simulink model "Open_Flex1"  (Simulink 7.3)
settings: Solver=ode4  StartTime=0.0  StopTime=20  RelTol=1e-3
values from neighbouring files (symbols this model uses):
  Ts = 0.04    [run.m]    (also in z2s_transf.m)
undefined symbols (not defined in the file or in its folder): Acts, Afls, Alfc, Apfc, Asz, Bcts, Bfls, Blfc, Bpfc, Bsz, Ccts, Cfls, Clfc, Cpfc, Csz, Dcts, Dfls, Dlfc, Dpfc, Dsz, TVC

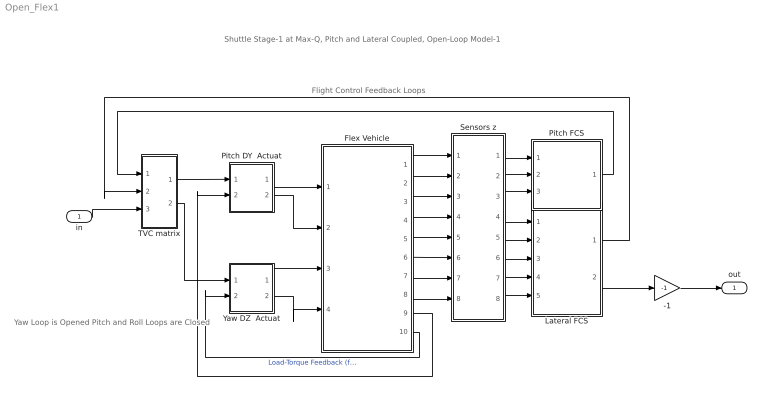
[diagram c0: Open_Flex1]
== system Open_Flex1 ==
  note: Shuttle Stage-1 at Max-Q, Pitch and Lateral Coupled, Open-Loop Model-1
  note: Yaw Loop is Opened Pitch and Roll Loops are Closed
  note: Flight Control Feedback Loops
  in : Inport  OutDataType=sfix(16)  OutScaling=2^0
  -1 : Gain  Gain=-1  ParameterDataType=sfix(16)  ParameterScaling=2^0  OutDataType=sfix(16)  OutScaling=2^0
  Flex Vehicle : Subsystem
  Lateral FCS : Subsystem
  Pitch DY  Actuat : Subsystem
  Pitch FCS : Subsystem
  Sensors z : Subsystem
  TVC matrix : Subsystem
  Yaw DZ  Actuat : Subsystem
  out : Outport  OutDataType=sfix(16)  OutScaling=2^0
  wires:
  TVC matrix/1(dy) -> Pitch DY  Actuat/1(dyc)
  TVC matrix/2(dz) -> Yaw DZ  Actuat/1(dzc)
  Pitch DY  Actuat/1(dy) -> Flex Vehicle/1(dy)
  Yaw DZ  Actuat/1(dz) -> Flex Vehicle/3(dz)
  Pitch DY  Actuat/2(dydd) -> Flex Vehicle/2(dydd)
  Yaw DZ  Actuat/2(dzdd) -> Flex Vehicle/4(dzdd)
  -1/1 -> out/1
  Flex Vehicle/10(TLz) -> Yaw DZ  Actuat/2(TLz)  "Load-Torque Feedback (ft-lb)"
  Flex Vehicle/9(TLy) -> Pitch DY  Actuat/2(TLy)
  Flex Vehicle/1(theta) -> Sensors z/1(thei)
  Sensors z/1(theo) -> Pitch FCS/1(theta)
  Flex Vehicle/2(q-flx) -> Sensors z/2(qi)
  Sensors z/2(qo) -> Pitch FCS/2(q)
  Flex Vehicle/3(Nz) -> Sensors z/3(Nzi)
  Sensors z/3(Nzo) -> Pitch FCS/3(Nz)
  Flex Vehicle/4(phi) -> Sensors z/4(phi)
  Sensors z/4(pho) -> Lateral FCS/1(phi-er)
  Flex Vehicle/5(psi) -> Sensors z/5("psi ")
  Sensors z/5(pso) -> Lateral FCS/2(psi-er)
  Flex Vehicle/6(p-flx) -> Sensors z/6(pi)
  Sensors z/6(po) -> Lateral FCS/3(p)
  Flex Vehicle/7(r-flx) -> Sensors z/7(ri)
  Sensors z/7(ro) -> Lateral FCS/4(r)
  Flex Vehicle/8(Ny) -> Sensors z/8(Nyi)
  Sensors z/8(Nyo) -> Lateral FCS/5(Ny)
  Lateral FCS/1(DP_TVC) -> TVC matrix/2(roll)
  in/1 -> TVC matrix/3(yaw)
  Lateral FCS/2(DR_TVC) -> -1/1
  Pitch FCS/1(DQ_TVC) -> TVC matrix/1(ptch)

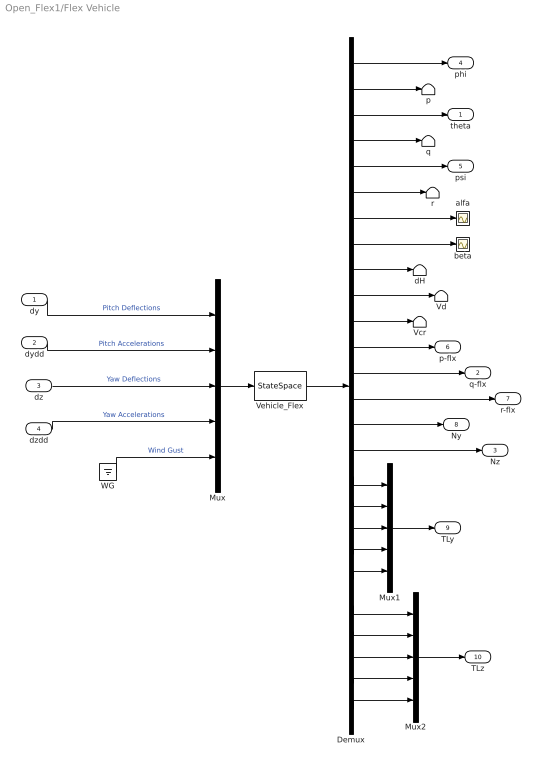
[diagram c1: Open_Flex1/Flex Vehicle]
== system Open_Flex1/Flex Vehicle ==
  dy : Inport  PortDimensions=5  OutDataType=sfix(16)  OutScaling=2^0
  dydd : Inport  Port=2  PortDimensions=5  OutDataType=sfix(16)  OutScaling=2^0
  dz : Inport  Port=3  PortDimensions=5  OutDataType=sfix(16)  OutScaling=2^0
  dzdd : Inport  Port=4  PortDimensions=5  OutDataType=sfix(16)  OutScaling=2^0
  Demux : Demux  Outputs=26
  Mux : Mux  Inputs="[5  5  5  5  1]"
  Mux1 : Mux  Inputs=5
  Mux2 : Mux  Inputs=5
  Vcr : Terminator
  Vd : Terminator
  Vehicle_Flex : StateSpace  A=Afls  B=Bfls  C=Cfls  D=Dfls
  WG : Ground
  alfa : Scope
  beta : Scope
  dH : Terminator
  p : Terminator
  q : Terminator
  r : Terminator
  theta : Outport  OutDataType=sfix(16)  OutScaling=2^0
  q-flx : Outport  Port=2  OutDataType=sfix(16)  OutScaling=2^0
  Nz : Outport  Port=3  OutDataType=sfix(16)  OutScaling=2^0
  phi : Outport  Port=4  OutDataType=sfix(16)  OutScaling=2^0
  psi : Outport  Port=5  OutDataType=sfix(16)  OutScaling=2^0
  p-flx : Outport  Port=6  OutDataType=sfix(16)  OutScaling=2^0
  r-flx : Outport  Port=7  OutDataType=sfix(16)  OutScaling=2^0
  Ny : Outport  Port=8  OutDataType=sfix(16)  OutScaling=2^0
  TLy : Outport  Port=9  OutDataType=sfix(16)  OutScaling=2^0
  TLz : Outport  Port=10  OutDataType=sfix(16)  OutScaling=2^0
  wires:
  Mux/1 -> Vehicle_Flex/1
  WG/1 -> Mux/5  "Wind Gust"
  dz/1 -> Mux/3  "Yaw Deflections"
  dydd/1 -> Mux/2  "Pitch Accelerations"
  dy/1 -> Mux/1  "Pitch Deflections"
  Demux/1 -> phi/1
  Demux/5 -> psi/1
  Demux/2 -> p/1
  Demux/6 -> r/1
  Demux/8 -> beta/1
  Demux/12 -> p-flx/1
  Demux/13 -> q-flx/1
  Demux/15 -> Ny/1
  Demux/3 -> theta/1
  Demux/4 -> q/1
  Demux/7 -> alfa/1
  Demux/11 -> Vcr/1
  Demux/10 -> Vd/1
  Demux/9 -> dH/1
  Demux/14 -> r-flx/1
  Demux/16 -> Nz/1
  dzdd/1 -> Mux/4  "Yaw Accelerations"
  Vehicle_Flex/1 -> Demux/1
  Demux/21 -> Mux1/5
  Demux/20 -> Mux1/4
  Demux/19 -> Mux1/3
  Demux/18 -> Mux1/2
  Demux/17 -> Mux1/1
  Demux/22 -> Mux2/1
  Demux/23 -> Mux2/2
  Demux/24 -> Mux2/3
  Demux/25 -> Mux2/4
  Demux/26 -> Mux2/5
  Mux1/1 -> TLy/1
  Mux2/1 -> TLz/1

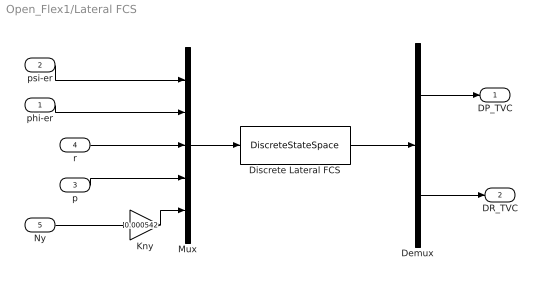
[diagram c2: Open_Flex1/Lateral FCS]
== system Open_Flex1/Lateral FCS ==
  phi-er : Inport  OutDataType=sfix(16)  OutScaling=2^0
  psi-er : Inport  Port=2  OutDataType=sfix(16)  OutScaling=2^0
  p : Inport  Port=3  OutDataType=sfix(16)  OutScaling=2^0
  r : Inport  Port=4  OutDataType=sfix(16)  OutScaling=2^0
  Ny : Inport  Port=5  OutDataType=sfix(16)  OutScaling=2^0
  Demux : Demux  Outputs=2
  Discrete Lateral FCS : DiscreteStateSpace  A=Alfc  B=Blfc  C=Clfc  D=Dlfc  SampleTime=Ts
  Kny : Gain  Gain=0.000542  ParameterDataType=sfix(16)  ParameterScaling=2^0  OutDataType=sfix(16)  OutScaling=2^0
  Mux : Mux  Inputs=5
  DP_TVC : Outport  OutDataType=sfix(16)  OutScaling=2^0
  DR_TVC : Outport  Port=2  OutDataType=sfix(16)  OutScaling=2^0
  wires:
  psi-er/1 -> Mux/1
  phi-er/1 -> Mux/2
  r/1 -> Mux/3
  Mux/1 -> Discrete Lateral FCS/1
  Discrete Lateral FCS/1 -> Demux/1
  Demux/1 -> DP_TVC/1
  Demux/2 -> DR_TVC/1
  p/1 -> Mux/4
  Ny/1 -> Kny/1
  Kny/1 -> Mux/5

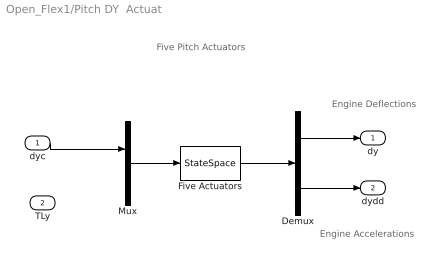
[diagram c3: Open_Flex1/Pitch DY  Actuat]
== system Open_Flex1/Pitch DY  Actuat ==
  note: Engine Accelerations
  note: Engine Deflections
  note: Five Pitch Actuators
  dyc : Inport  OutDataType=sfix(16)  OutScaling=2^0
  TLy : Inport  Port=2  OutDataType=sfix(16)  OutScaling=2^0
  Demux : Demux  Outputs=[5, 5]
  Five Actuators : StateSpace  A=Acts  B=Bcts  C=Ccts  D=Dcts
  Mux : Mux  Inputs="[5  5]"
  dy : Outport  OutDataType=sfix(16)  OutScaling=2^0
  dydd : Outport  Port=2  OutDataType=sfix(16)  OutScaling=2^0
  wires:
  Mux/1 -> Five Actuators/1
  dyc/1 -> Mux/1
  Five Actuators/1 -> Demux/1
  Demux/1 -> dy/1
  Demux/2 -> dydd/1

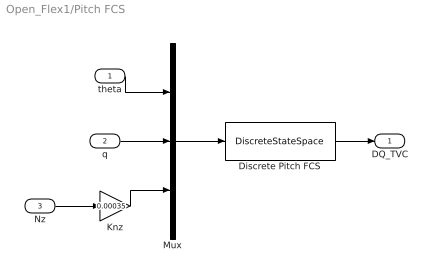
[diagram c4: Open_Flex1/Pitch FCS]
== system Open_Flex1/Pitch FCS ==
  theta : Inport  OutDataType=sfix(16)  OutScaling=2^0
  q : Inport  Port=2  OutDataType=sfix(16)  OutScaling=2^0
  Nz : Inport  Port=3  OutDataType=sfix(16)  OutScaling=2^0
  Discrete Pitch FCS : DiscreteStateSpace  A=Apfc  B=Bpfc  C=Cpfc  D=Dpfc  SampleTime=Ts
  Knz : Gain  Gain=0.00035  ParameterDataType=sfix(16)  ParameterScaling=2^0  OutDataType=sfix(16)  OutScaling=2^0
  Mux : Mux  Inputs=3
  DQ_TVC : Outport  OutDataType=sfix(16)  OutScaling=2^0
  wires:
  Mux/1 -> Discrete Pitch FCS/1
  Nz/1 -> Knz/1
  q/1 -> Mux/2
  theta/1 -> Mux/1
  Discrete Pitch FCS/1 -> DQ_TVC/1
  Knz/1 -> Mux/3

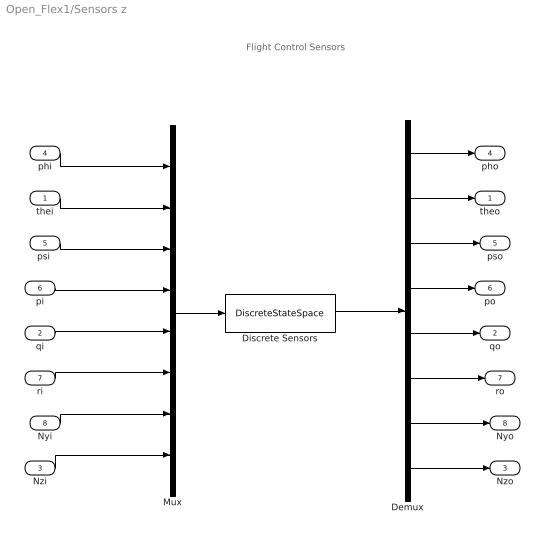
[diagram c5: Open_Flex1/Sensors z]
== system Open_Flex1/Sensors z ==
  note: Flight Control Sensors
  thei : Inport  PortDimensions=1  OutDataType=sfix(16)  OutScaling=2^0
  qi : Inport  Port=2  PortDimensions=1  OutDataType=sfix(16)  OutScaling=2^0
  Nzi : Inport  Port=3  PortDimensions=1  OutDataType=sfix(16)  OutScaling=2^0
  phi : Inport  Port=4  PortDimensions=1  OutDataType=sfix(16)  OutScaling=2^0
  "psi " : Inport  Port=5  PortDimensions=1  OutDataType=sfix(16)  OutScaling=2^0
  pi : Inport  Port=6  PortDimensions=1  OutDataType=sfix(16)  OutScaling=2^0
  ri : Inport  Port=7  PortDimensions=1  OutDataType=sfix(16)  OutScaling=2^0
  Nyi : Inport  Port=8  PortDimensions=1  OutDataType=sfix(16)  OutScaling=2^0
  Demux : Demux  Outputs=8
  Discrete Sensors : DiscreteStateSpace  A=Asz  B=Bsz  C=Csz  D=Dsz  SampleTime=Ts
  Mux : Mux  Inputs=8
  theo : Outport  OutDataType=sfix(16)  OutScaling=2^0
  qo : Outport  Port=2  OutDataType=sfix(16)  OutScaling=2^0
  Nzo : Outport  Port=3  OutDataType=sfix(16)  OutScaling=2^0
  pho : Outport  Port=4  OutDataType=sfix(16)  OutScaling=2^0
  pso : Outport  Port=5  OutDataType=sfix(16)  OutScaling=2^0
  po : Outport  Port=6  OutDataType=sfix(16)  OutScaling=2^0
  ro : Outport  Port=7  OutDataType=sfix(16)  OutScaling=2^0
  Nyo : Outport  Port=8  OutDataType=sfix(16)  OutScaling=2^0
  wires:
  Mux/1 -> Discrete Sensors/1
  Discrete Sensors/1 -> Demux/1
  phi/1 -> Mux/1
  thei/1 -> Mux/2
  "psi "/1 -> Mux/3
  pi/1 -> Mux/4
  qi/1 -> Mux/5
  ri/1 -> Mux/6
  Nyi/1 -> Mux/7
  Nzi/1 -> Mux/8
  Demux/1 -> pho/1
  Demux/2 -> theo/1
  Demux/3 -> pso/1
  Demux/4 -> po/1
  Demux/5 -> qo/1
  Demux/6 -> ro/1
  Demux/7 -> Nyo/1
  Demux/8 -> Nzo/1

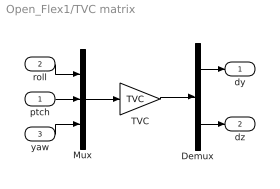
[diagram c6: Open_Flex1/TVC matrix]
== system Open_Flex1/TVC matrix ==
  ptch : Inport  OutDataType=sfix(16)  OutScaling=2^0
  roll : Inport  Port=2  OutDataType=sfix(16)  OutScaling=2^0
  yaw : Inport  Port=3  OutDataType=sfix(16)  OutScaling=2^0
  Demux : Demux  Outputs="[5  5]"
  Mux : Mux  Inputs=3
  TVC : Gain  Gain=TVC  Multiplication=Matrix(K*u) (u vector)  ParameterDataType=sfix(16)  ParameterScaling=2^0  OutDataType=sfix(16)  OutScaling=2^0
  dy : Outport  OutDataType=sfix(16)  OutScaling=2^0
  dz : Outport  Port=2  OutDataType=sfix(16)  OutScaling=2^0
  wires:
  TVC/1 -> Demux/1
  Mux/1 -> TVC/1
  roll/1 -> Mux/1
  Demux/1 -> dy/1
  ptch/1 -> Mux/2
  Demux/2 -> dz/1
  yaw/1 -> Mux/3

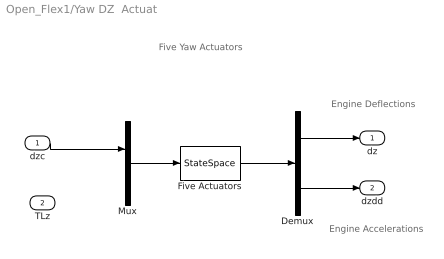
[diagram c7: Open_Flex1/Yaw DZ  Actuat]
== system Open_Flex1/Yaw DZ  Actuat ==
  note: Engine Accelerations
  note: Engine Deflections
  note: Five Yaw Actuators
  dzc : Inport  OutDataType=sfix(16)  OutScaling=2^0
  TLz : Inport  Port=2  OutDataType=sfix(16)  OutScaling=2^0
  Demux : Demux  Outputs=[5, 5]
  Five Actuators : StateSpace  A=Acts  B=Bcts  C=Ccts  D=Dcts
  Mux : Mux  Inputs="[5  5]"
  dz : Outport  OutDataType=sfix(16)  OutScaling=2^0
  dzdd : Outport  Port=2  OutDataType=sfix(16)  OutScaling=2^0
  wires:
  Mux/1 -> Five Actuators/1
  dzc/1 -> Mux/1
  Five Actuators/1 -> Demux/1
  Demux/1 -> dz/1
  Demux/2 -> dzdd/1
